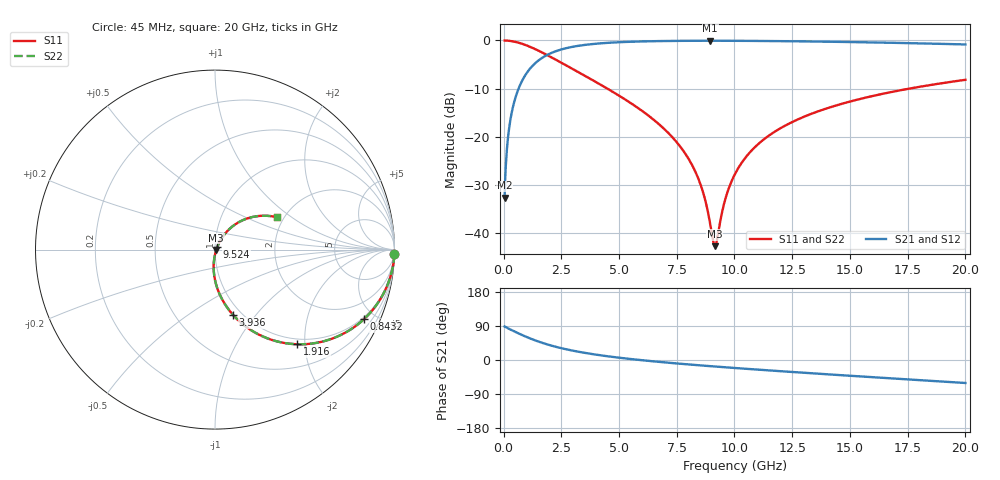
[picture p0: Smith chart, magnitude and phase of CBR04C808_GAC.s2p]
! S-parameter model data by Modelithics Inc.  support@modelithics.com 813-866-6335  Tampa FL USA
! S-Parameter data specifications:
! Substrate: 20-mil Rogers 4350B, substrate thickness, H=0.508mm, Dielectric constant, Er=3.75
! PCB Mounting Pad Footprint: Pad width, PadW=0.52mm , Pad length, PadL=0.52mm , Pad gap, PadG (edge-to-edge)=0.28mm , Reference planes=1.32mm apart
#  GHz  S  MA  R 50
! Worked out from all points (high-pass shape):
!   801 points, 45 MHz to 20 GHz, reference 50 ohm
!   highest |S21| = -0.07 dB at 8.95 GHz (marker M1); lowest = -32.7 dB at 45 MHz (marker M2)
!   |S21| within 3 dB of the highest: 1.868 GHz to end of sweep
!   lowest |S11| = -42.8 dB at 9.149 GHz (marker M3), VSWR 1.01, Z = 50.7 - j0.24 ohm
!   |S11| at or under -10 dB: 4.488 GHz to 17.59 GHz (13.1 GHz wide, 119 % of centre)
!   |S22| runs from -42.8 to 0.0 dB; largest |S21 - S12| = 0
!   S11 on the Smith chart (normalised r, x): 45 MHz: 1, -81; 843.2 MHz: 0.90, -4.33; 1.916 GHz: 0.90, -1.84; 3.936 GHz: 0.91, -0.77; 9.524 GHz: 1.03, +0.03; 20 GHz: 1.84, +0.78
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0.045  0.9997 -1.4  0.02319 88.5  0.02319 88.5  0.9997 -1.4
0.194662  0.9945 -6.1  0.09938 83.6  0.09938 83.6  0.9945 -6.1
0.319381  0.986 -9.9  0.1613 79.8  0.1613 79.8  0.986 -9.9
0.543875  0.9621 -16.6  0.2681 73.2  0.2681 73.2  0.9621 -16.6
0.8432  0.9161 -25.0  0.3972 64.8  0.3972 64.8  0.9161 -25.0
1.342075  0.8182 -37.4  0.5717 52.4  0.5717 52.4  0.8182 -37.4
1.915781  0.6986 -49.0  0.7122 40.7  0.7122 40.7  0.6986 -49.0
3.387462  0.4473 -69.3  0.8901 20.2  0.8901 20.2  0.4473 -69.3
3.936225  0.377 -74.6  0.9216 14.7  0.9216 14.7  0.377 -74.6
6.704981  0.1362 -92.2  0.9844 -4.8  0.9844 -4.8  0.1362 -92.2
7.578012  0.08289 -95.0  0.9898 -9.5  0.9898 -9.5  0.08289 -95.0
8.201606  0.04863 -94.6  0.9918 -12.7  0.9918 -12.7  0.04863 -94.6
8.62565  0.02704 -89.7  0.9924 -14.7  0.9924 -14.7  0.02704 -89.7
8.949919  0.01225 -70.4  0.9925 -16.3  0.9925 -16.3  0.01225 -70.4
9.149469  0.007263 -19.1  0.9924 -17.2  0.9924 -17.2  0.007263 -19.1
9.249244  0.008601 14.2  0.9924 -17.6  0.9924 -17.6  0.008601 14.2
9.523625  0.01897 48.0  0.9921 -18.9  0.9921 -18.9  0.01897 48.0
10.0225  0.04088 58.1  0.9912 -21.1  0.9912 -21.1  0.04088 58.1
11.26969  0.09357 58.4  0.9871 -26.5  0.9871 -26.5  0.09357 58.4
13.36496  0.1739 51.9  0.9753 -35.1  0.9753 -35.1  0.1739 51.9
16.68248  0.2873 39.8  0.9469 -48.1  0.9469 -48.1  0.2873 39.8
20  0.3897 27.6  0.9085 -60.7  0.9085 -60.7  0.3897 27.6
